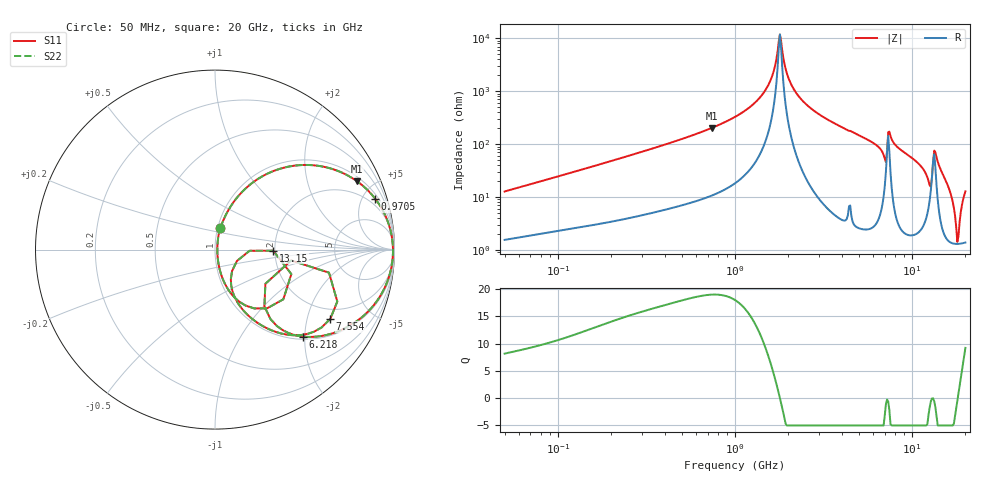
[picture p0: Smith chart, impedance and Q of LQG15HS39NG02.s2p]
!Murata Part Number: LQG15HS39NG02
!These Parameters are Measured in Series Mode Connection
!  o--[Z]--o
!Port1  Port2
!  o-------o
!Freq. Start=50[MHz] Stop=20[GHz], 401[Steps]
# Hz S RI R 50
!Freq.(Hz) S11(Real) S11(Imag) S21(Real) S21(Imag) S12(Real) S12(Imag) S22(Real) S22(Imag)
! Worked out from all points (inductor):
!   401 points, 50 MHz to 20 GHz, reference 50 ohm
!   read as one part in series: L = 39.6 nH near 51.52 MHz
!   highest Q = 19 at 741.1 MHz (marker M1), where L = 43.6 nH
!   self-resonance near 1.793 GHz
!   S11 on the Smith chart (normalised r, x): 50 MHz: 1.03, +0.25; 970.5 MHz: 1.34, +6.18; 6.218 GHz: 1.06, -1.97; 7.554 GHz: 1.58, -2.79; 13.15 GHz: 1.96, -0.03; 20 GHz: 1.03, +0.25
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5e7  0.0303 0.1207  0.9697 -0.1207  0.9697 -0.1207  0.0303 0.1207
1.364002e8  0.117 0.2828  0.883 -0.2828  0.883 -0.2828  0.117 0.2828
3.721004e8  0.4518 0.4687  0.5482 -0.4687  0.5482 -0.4687  0.4518 0.4687
7.411344e8  0.7927 0.3799  0.2073 -0.3799  0.2073 -0.3799  0.7927 0.3799
9.70487e8  0.893 0.2829  0.107 -0.2829  0.107 -0.2829  0.893 0.2829
1e9  0.9021 0.2707  0.0979 -0.2707  0.0979 -0.2707  0.9021 0.2707
1.498439e9  0.9821 0.0877  0.0179 -0.0877  0.0179 -0.0877  0.9821 0.0877
1.793498e9  0.9916 0.000168  0.00838 -0.000168  0.00838 -0.000168  0.9916 0.000168
2.083303e9  0.987 -0.074  0.013 0.074  0.013 0.074  0.987 -0.074
2.728004e9  0.9478 -0.2075  0.0522 0.2075  0.0522 0.2075  0.9478 -0.2075
6.217679e9  0.4918 -0.4849  0.5082 0.4849  0.5082 0.4849  0.4918 -0.4849
6.905011e9  0.3091 -0.3872  0.6909 0.3872  0.6909 0.3872  0.3091 -0.3872
7.442007e9  0.6815 -0.2893  0.3185 0.2893  0.3185 0.2893  0.6815 -0.2893
7.554318e9  0.6421 -0.3863  0.3579 0.3863  0.3579 0.3863  0.6421 -0.3863
8.516016e9  0.3984 -0.4733  0.6016 0.4733  0.6016 0.4733  0.3984 -0.4733
1.183995e10  0.1051 -0.2539  0.8949 0.2539  0.8949 0.2539  0.1051 -0.2539
1.257102e10  0.0952 -0.119  0.9048 0.119  0.9048 0.119  0.0952 -0.119
1.314879e10  0.3248 -0.00605  0.6752 0.00605  0.6752 0.00605  0.3248 -0.00605
1.375312e10  0.2897 -0.3275  0.7103 0.3275  0.7103 0.3275  0.2897 -0.3275
1.573793e10  0.0456 -0.1691  0.9544 0.1691  0.9544 0.1691  0.0456 -0.1691
1.800918e10  0.0129 -0.00552  0.9871 0.00552  0.9871 0.00552  0.0129 -0.00552
2e10  0.0289 0.1218  0.9711 -0.1218  0.9711 -0.1218  0.0289 0.1218
